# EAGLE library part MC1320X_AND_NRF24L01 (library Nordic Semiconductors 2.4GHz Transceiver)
With this Device, it is possible to use the NRF24L01 or the MC1320x 802.15.4 transceiver
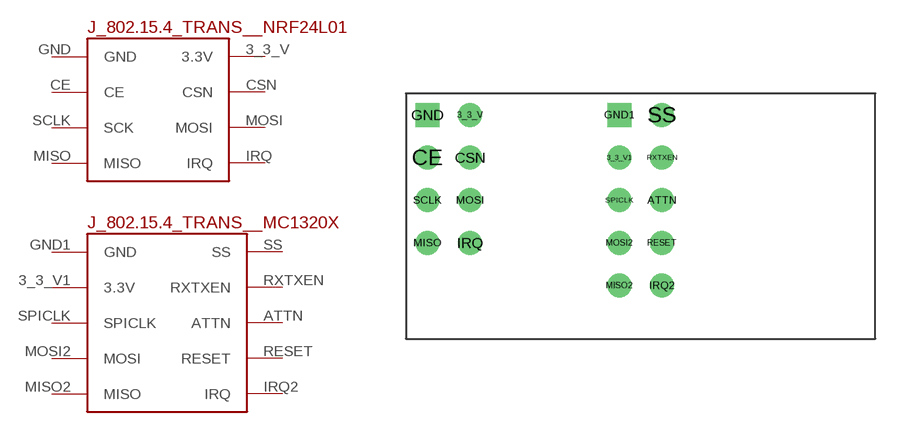
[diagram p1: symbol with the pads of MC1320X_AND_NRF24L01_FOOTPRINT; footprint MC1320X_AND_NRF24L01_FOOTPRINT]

Designator prefix J_802.15.4_TRANS_; gates _MC1320X=MC1320X_RF_DAUGHTER_CARD _NRF24L01=NRF24L01_MODULE_SCHEMATIC

## MC1320X_AND_NRF24L01  [MC1320X_AND_NRF24L01_FOOTPRINT]
3_3_V  _NRF24L01:3.3V
3_3_V1  _MC1320X:3.3V
ATTN  _MC1320X:ATTN
CE  _NRF24L01:CE
CSN  _NRF24L01:CSN
GND  _NRF24L01:GND
GND1  _MC1320X:GND
IRQ  _NRF24L01:IRQ
IRQ2  _MC1320X:IRQ
MISO  _NRF24L01:MISO
MISO2  _MC1320X:MISO
MOSI  _NRF24L01:MOSI
MOSI2  _MC1320X:MOSI
RESET  _MC1320X:RESET
RXTXEN  _MC1320X:RXTXEN
SCLK  _NRF24L01:SCK
SPICLK  _MC1320X:SPICLK
SS  _MC1320X:SS

## Footprint MC1320X_AND_NRF24L01_FOOTPRINT (pad centres in mm)
With this Footprint, it is possible to use the NRF24L01 or the MC1320x 802.15.4 transceiver
drill 0.9 pad 1.422: 3_3_V -11.43,6.35; 3_3_V1 -2.54,3.81; ATTN 0,1.27; CE -13.97,3.81; CSN -11.43,3.81; IRQ -11.43,-1.27; IRQ2 0,-3.81; MISO -13.97,-1.27; MISO2 -2.54,-3.81; MOSI -11.43,1.27; MOSI2 -2.54,-1.27; RESET 0,-1.27; RXTXEN 0,3.81; SCLK -13.97,1.27; SPICLK -2.54,1.27; SS 0,6.35
drill 0.9 pad 1.422 square: GND -13.97,6.35; GND1 -2.54,6.35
